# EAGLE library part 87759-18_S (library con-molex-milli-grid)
HEADER
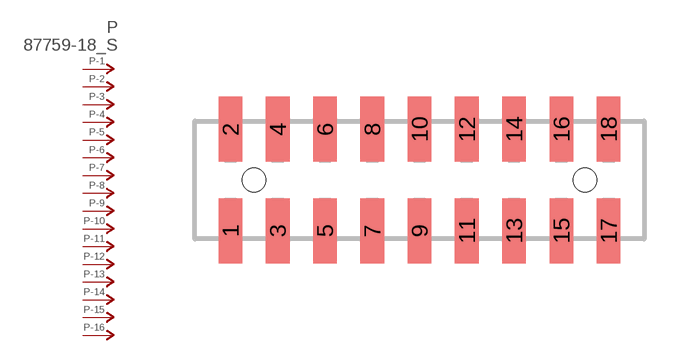
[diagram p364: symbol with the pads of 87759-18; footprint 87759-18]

Designator prefix P; gates -1=P-NV -2=P-N -3=P-N -4=P-N -5=P-N -6=P-N -7=P-N -8=P-N -9=P-N -10=P-N -11=P-N -12=P-N -13=P-N -14=P-N -15=P-N -16=P-N -17=P-N -18=P-N

## 87759-18_S  [87759-18]
1  -1:P  pas
2  -2:P  pas
3  -3:P  pas
4  -4:P  pas
5  -5:P  pas
6  -6:P  pas
7  -7:P  pas
8  -8:P  pas
9  -9:P  pas
10  -10:P  pas
11  -11:P  pas
12  -12:P  pas
13  -13:P  pas
14  -14:P  pas
15  -15:P  pas
16  -16:P  pas
17  -17:P  pas
18  -18:P  pas

## Footprint 87759-18 (pad centres in mm)
HEADER SMD Dual Row, Vertical
smd 1 x 2.75: 1 -8,-2.15; 2 -8,2.15; 3 -6,-2.15; 4 -6,2.15; 5 -4,-2.15; 6 -4,2.15; 7 -2,-2.15; 8 -2,2.15; 9 0,-2.15; 10 0,2.15; 11 2,-2.15; 12 2,2.15; 13 4,-2.15; 14 4,2.15; 15 6,-2.15; 16 6,2.15; 17 8,-2.15; 18 8,2.15
hole 1 at -7,0
hole 1 at 7,0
